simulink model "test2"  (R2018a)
settings: Solver=FixedStepAuto  StartTime=0.0  StopTime=inf  FixedStep=0.02  RelTol=1e-3  EnableMultiTasking=on
undefined symbols (not defined in the file or in its folder): bit, C, CCAN, identifier, Radius_Calculation_ROS_2017b, Srikanth_TA, Standard
libraries: canmsglib x2, PCANLibrary x2

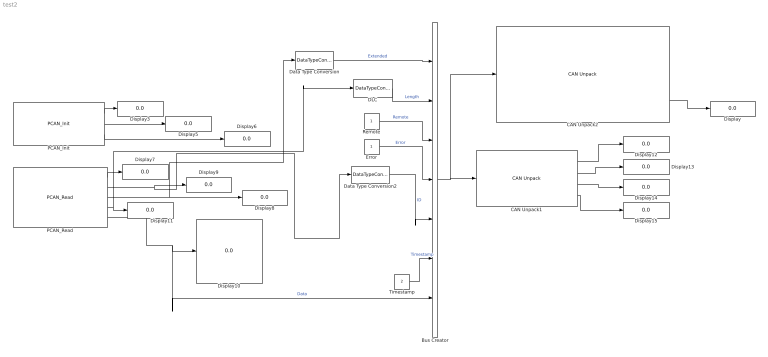
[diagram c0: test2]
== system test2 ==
  Bus Creator : BusCreator  Inputs=7  OutDataTypeStr=Bus: CAN_MESSAGE_BUS
  CAN Unpack1 : canmsglib/CAN Unpack  CANdbFile=C:\Srikanth_TA\20180903\Radius_Calculation_ROS_2017b\CCAN.dbc  MsgList=WHL_SPD11  MsgName=WHL_SPD11  MsgIDType=Standard (11-bit identifier)  MsgIdentifier=902  MsgLength=8  SignalInfo=WHL_SPD_FL$0$14$1$2$1$0$3.125000e-02$0$0$5.119688e+02$#WHL_SPD_FR$16$14$1$2$1$0$3.125000e-02$0$0$5.119688e+02$#WHL_SPD_RL$32$14$1$2$1$0$3.125000e-02$0$0$5.119688e+02$#WHL_SPD_RR$48$14$1$2$1$0$3.125000e-02$0$0$5.119688e+02$#  NSignals=4  IDPort=off  TimestampPort=off  ErrorPort=off  RemotePort=off  LengthPort=off  StatusPort=off  StartBits=str2num('[int32(0);int32(16);int32(32);int32(48)]')  SignalSizes=str2num('[int32(14);int32(14);int32(14);int32(14)]')  ByteOrders=str2num('[int32(1);int32(1);int32(1);int32(1)]')  DataTypes=str2num('[int32(2);int32(2);int32(2);int32(2)]')  MultiplexTypes=str2num('[int32(1);int32(1);int32(1);int32(1)]')  MultiplexValues=str2num('[double(0);double(0);double(0);double(0)]')  Factors=str2num('[double(3.125000e-02);double(3.125000e-02);double(3.125000e-02);double(3.125000e-02)]')  Offsets=str2num('[double(0);double(0);double(0);double(0)]')  Minimums=str2num('[double(0);double(0);double(0);double(0)]')  Maximums=str2num('[double(5.119688e+02);double(5.119688e+02);double(5.119688e+02);double(5.119688e+02)]')  ApplyMinMax=off
  CAN Unpack2 : canmsglib/CAN Unpack  CANdbFile=C:\Srikanth_TA\20180903\Radius_Calculation_ROS_2017b\CCAN.dbc  MsgList=ESP12  MsgName=ESP12  MsgIDType=Standard (11-bit identifier)  MsgIdentifier=544  MsgLength=7  SignalInfo=CYL_PRES$26$12$1$2$1$0$1.000000e-01$0$0$4.095000e+02$#CYL_PRES_DIAG$39$1$1$2$1$0$1$0$0$1$#CYL_PRES_STAT$38$1$1$2$1$0$1$0$0$1$#LAT_ACCEL$0$11$1$2$1$0$1.000000e-02$-1.023000e+01$-1.023000e+01$1.024000e+01$#LAT_ACCEL_DIAG$12$1$1$2$1$0$1$0$0$1$#LAT_ACCEL_STAT$11$1$1$2$1$0$1$0$0$1$#LONG_ACCEL$13$11$1$2$1$0$1.000000e-02$-1.023000e+01$-1.023000e+01$1.024000e+01$#LONG_ACCEL_DIAG$25$1$1$2$1$0$1$0$0$1$#LONG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  NSignals=12  IDPort=off  TimestampPort=off  ErrorPort=off  RemotePort=off  LengthPort=off  StatusPort=off  StartBits=str2num('[int32(26);int32(39);int32(38);int32(0);int32(12);int32(11);int32(13);int32(25);int32(24);int32(40);int32(54);int32(53)]')  SignalSizes=str2num('[int32(12);int32(1);int32(1);int32(11);int32(1);int32(1);int32(11);int32(1);int32(1);int32(13);int32(1);int32(1)]')  ByteOrders=str2num('[int32(1);int32(1);int32(1);int32(1);int32(1);int32(1);int32(1);int32(1);int32(1);int32(1);int32(1);int32(1)]')  DataTypes=str2num('[int32(2);int32(2);int32(2);int32(2);int32(2);int32(2);int32(2);int32(2);int32(2);int32(2);int32(2);int32(2)]')  MultiplexTypes=str2num('[int32(1);int32(1);int32(1);int32(1);int32(1);int32(1);int32(1);int32(1);int32(1);int32(1);int32(1);int32(1)]')  MultiplexValues=str2num('[double(0);double(0);double(0);double(0);double(0);double(0);double(0);double(0);double(0);double(0);double(0);double(0)]')  Factors=str2num('[double(1.000000e-01);double(1);double(1);double(1.000000e-02);double(1);double(1);double(1.000000e-02);double(1);double(1);double(1.000000e-02);double(1);double(1)]')  Offsets=str2num('[double(0);double(0);double(0);double(-1.023000e+01);double(0);double(0);double(-1.023000e+01);double(0);double(0);double(-4.095000e+01);double(0);double(0)]')  Minimums=str2num('[double(0);double(0);double(0);double(-1.023000e+01);double(0);double(0);double(-1.023000e+01);double(0);double(0);double(-4.095000e+01);double(0);double(0)]')  Maximums=str2num('[double(4.095000e+02);double(1);double(1);double(1.024000e+01);double(1);double(1);double(1.024000e+01);double(1);double(1);double(4.096000e+01);double(1);double(1)]')  ApplyMinMax=off
  DLC : DataTypeConversion  OutDataTypeStr=uint8
  Data Type Conversion : DataTypeConversion  OutDataTypeStr=uint8
  Data Type Conversion2 : DataTypeConversion  OutDataTypeStr=uint32
  Display{,3,5..15} (13 alike) : Display
  Error : Constant  OutDataTypeStr=uint8
  PCAN_Init : PCANLibrary/PCAN_Init  pcanusb=PCAN_USBBUS1  Initvar='1C'  MsgFormat=0  FromID='00'  ToID='7FF'
  PCAN_Read : PCANLibrary/PCAN_Read  PcanUsbChannel=PCAN_USBBUS1
  Remote : Constant  OutDataTypeStr=uint8
  Timestamp : Constant  Value=2  OutDataTypeStr=double
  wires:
  PCAN_Read/3 -> Data Type Conversion/1, Display8/1
  PCAN_Init/3 -> Display6/1
  PCAN_Read/1 -> Display7/1
  PCAN_Init/2 -> Display5/1
  PCAN_Init/1 -> Display3/1
  Remote/1 -> Bus Creator/3  "Remote"
  Timestamp/1 -> Bus Creator/6  "Timestamp"
  DLC/1 -> Bus Creator/2  "Length"
  Data Type Conversion2/1 -> Bus Creator/5  "ID"
  Error/1 -> Bus Creator/4  "Error"
  Data Type Conversion/1 -> Bus Creator/1  "Extended"
  PCAN_Read/4 -> DLC/1, Display11/1
  PCAN_Read/2 -> Data Type Conversion2/1, Display9/1
  PCAN_Read/5 -> Bus Creator/7, Display10/1  "Data"
  CAN Unpack1/4 -> Display15/1
  CAN Unpack1/2 -> Display13/1
  CAN Unpack1/1 -> Display12/1
  CAN Unpack1/3 -> Display14/1
  Bus Creator/1 -> CAN Unpack2/1, CAN Unpack1/1
  CAN Unpack2/10 -> Display/1
